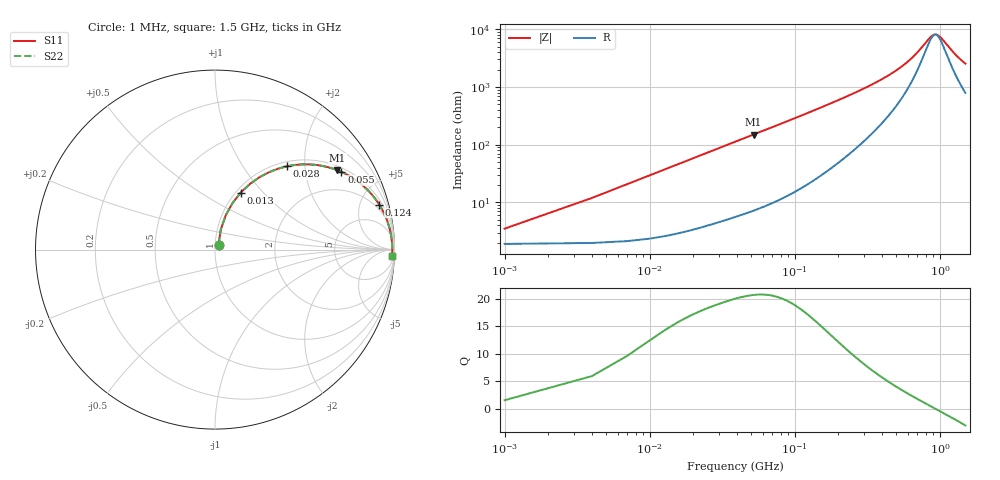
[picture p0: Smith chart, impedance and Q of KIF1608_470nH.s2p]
# MHz S RI R 50
!Freq ReS11 ImS11 ReS21 ImS21 ReS12 ImS12 ReS22 ImS22
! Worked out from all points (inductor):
!   501 points, 1 MHz to 1.5 GHz, reference 50 ohm
!   read as one part in series: L = 467 nH near 7 MHz
!   highest Q = 20.7 at 52 MHz (marker M1), where L = 456 nH
!   self-resonance near 931.3 MHz
!   S11 on the Smith chart (normalised r, x): 1 MHz: 1.04, +0.06; 13 MHz: 1.05, +0.76; 28 MHz: 1.09, +1.62; 55 MHz: 1.15, +3.15; 124 MHz: 1.42, +7.15; 1.5 GHz: 17, -48
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1  0.0196 0.0283  0.9804 -0.0283  0.9804 -0.0283  0.0196 0.0283
4  0.0324 0.1118  0.9676 -0.1118  0.9676 -0.1118  0.0324 0.1118
10  0.0973 0.2589  0.9027 -0.2589  0.9027 -0.2589  0.0973 0.2589
13  0.1435 0.3177  0.8565 -0.3177  0.8565 -0.3177  0.1435 0.3177
19  0.2478 0.4032  0.7522 -0.4032  0.7522 -0.4032  0.2478 0.4032
28  0.4021 0.4645  0.5979 -0.4645  0.5979 -0.4645  0.4021 0.4645
40  0.567 0.4713  0.433 -0.4713  0.433 -0.4713  0.567 0.4713
52  0.6821 0.4422  0.3179 -0.4422  0.3179 -0.4422  0.6821 0.4422
55  0.7046 0.4328  0.2954 -0.4328  0.2954 -0.4328  0.7046 0.4328
82  0.8348 0.3473  0.1652 -0.3473  0.1652 -0.3473  0.8348 0.3473
124  0.9151 0.251  0.0849 -0.251  0.0849 -0.251  0.9151 0.251
181  0.9535 0.1761  0.0465 -0.1761  0.0465 -0.1761  0.9535 0.1761
253  0.9712 0.1237  0.0288 -0.1237  0.0288 -0.1237  0.9712 0.1237
349  0.9802 0.0841  0.0198 -0.0841  0.0198 -0.0841  0.9802 0.0841
502  0.9853 0.0485  0.0147 -0.0485  0.0147 -0.0485  0.9853 0.0485
751  0.9875 0.016  0.0125 -0.016  0.0125 -0.016  0.9875 0.016
838  0.9878 0.00782  0.0122 -0.00782  0.0122 -0.00782  0.9878 0.00782
895  0.9878 0.00294  0.0122 -0.00294  0.0122 -0.00294  0.9878 0.00294
946  0.9878 -0.00115  0.0122 0.00115  0.0122 0.00115  0.9878 -0.00115
1003  0.9878 -0.00548  0.0122 0.00548  0.0122 0.00548  0.9878 -0.00548
1252  0.9874 -0.0222  0.0126 0.0222  0.0126 0.0222  0.9874 -0.0222
1500  0.9865 -0.0365  0.0135 0.0365  0.0135 0.0365  0.9865 -0.0365
